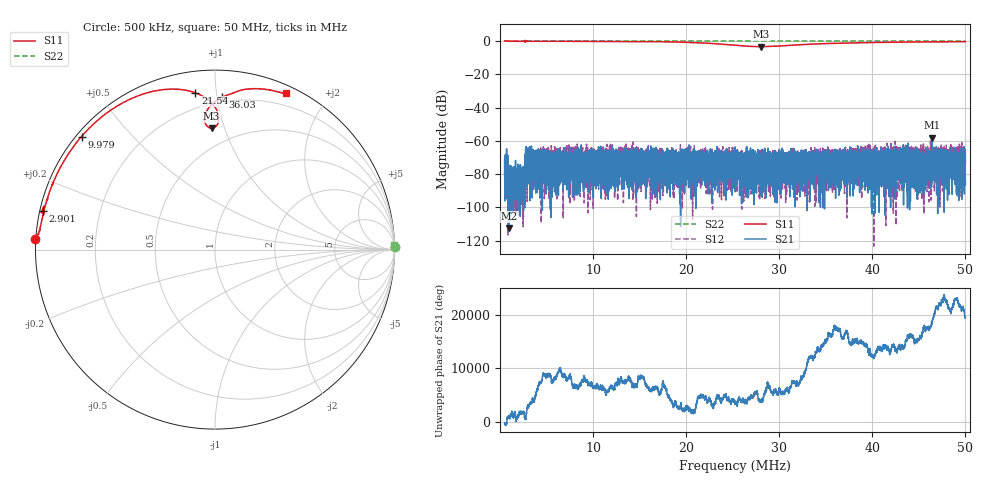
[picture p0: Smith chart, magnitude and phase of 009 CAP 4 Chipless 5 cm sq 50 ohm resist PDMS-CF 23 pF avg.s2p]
!  26/06/2025  15:42:23
! Ref Plane: 0.000 mm
# MHZ S MA R  50
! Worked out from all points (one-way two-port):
!   10001 points, 500 kHz to 50 MHz, reference 50 ohm
!   highest |S21| = -58.03 dB at 46.41 MHz (marker M1); lowest = -112.6 dB at 995 kHz (marker M2)
!   lowest |S11| = -3.4 dB at 28.09 MHz (marker M3), VSWR 5.18, Z = 18.1 + j45.2 ohm
!   |S11| at or under -10 dB: nowhere
!   |S22| runs from -0.2 to 0.3 dB; largest |S21 - S12| = 0.0012
!   S11 on the Smith chart (normalised r, x): 500 kHz: -0.00, +0.03; 2.901 MHz: 0.01, +0.11; 9.979 MHz: 0.01, +0.37; 21.54 MHz: 0.11, +0.88; 36.03 MHz: 0.17, +1.03; 50 MHz: 0.08, +1.55
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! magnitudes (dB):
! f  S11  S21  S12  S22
! 500 kHz  0.0  -71.4  -81.4  0.0
! 995 kHz  -0.1  -112.6  -95.2  0.0
! 2.45 MHz  -0.2  -82.5  -94.1  0.0
! 2.901 MHz  -0.1  -67.7  -67.7  0.0
! 8.752 MHz  -0.2  -65.4  -71.1  0.0
! 9.979 MHz  -0.2  -79.3  -78.8  0.0
! 15.54 MHz  -0.3  -70.0  -71.5  0.0
! 16 MHz  -0.4  -69.7  -66.2  0.0
! 17 MHz  -0.4  -83.3  -88.4  0.0
! 19.69 MHz  -0.7  -71.1  -74.6  0.0
! 21.54 MHz  -1.1  -76.7  -65.5  0.0
! 25.25 MHz  -2.6  -76.5  -85.4  0.0
! 28.09 MHz  -3.4  -79.0  -69.5  0.0
! 28.64 MHz  -3.4  -77.2  -80.9  0.0
! 33.5 MHz  -1.9  -72.8  -70.7  0.0
! 36.03 MHz  -1.4  -67.6  -72.5  0.0
! 41.75 MHz  -0.8  -77.8  -74.1  0.0
! 45.39 MHz  -0.6  -73.0  -71.0  0.0
! 46.41 MHz  -0.5  -58.0  -64.0  0.0
! 47.89 MHz  -0.5  -72.5  -74.2  0.0
! 49.68 MHz  -0.4  -70.5  -71.1  0.0
! 50 MHz  -0.4  -85.3  -74.8  0.0
